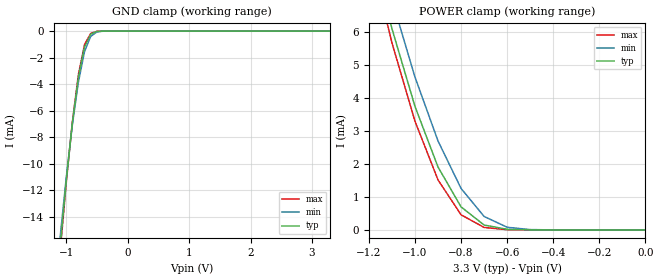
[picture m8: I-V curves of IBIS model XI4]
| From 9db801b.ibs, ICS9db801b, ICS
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|   Model XI4
[Model]   XI4
Model_type   Input
Polarity   Non-Inverting
Vinl =   0.175V
Vinh =   0.525V
C_comp   3.40pF   2.85pF   3.95pF
[Temperature Range]   25.00   71.00   1.00
[Voltage Range]   3.30V   3.00V   3.70V
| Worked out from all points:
|   GND clamp passes 1 mA (typ) near -0.68 V on its own axis
|   POWER clamp passes 1 mA (typ) near -0.82 V on its own axis
[GND_clamp]
| voltage   I(typ)   I(min)   I(max)
-3.3V     -160mA     -150mA     -160mA
-1.1V     -16.38mA   -15.67mA   -16.85mA
-1V       -11.38mA   -11.14mA   -11.54mA
-900mV    -6.99mA    -7.13mA    -6.92mA
-800mV    -3.48mA    -3.84mA    -3.27mA
-700mV    -1.2mA     -1.54mA    -1.01mA
-600mV    -240uA     -400uA     -170uA
-500mV    -29.28uA   -66.42uA   -17.31uA
-400mV    -2.53uA    -8.31uA    -1.16uA
3.3V      160pA      130nA      110pA
[POWER_clamp]
| voltage   I(typ)   I(min)   I(max)
-3.3V     130mA      120mA      140mA
-1.2V     8.92mA     9.69mA     8.55mA
-1.1V     6.11mA     6.99mA     5.68mA
-1V       3.75mA     4.64mA     3.3mA
-900mV    1.91mA     2.7mA      1.52mA
-800mV    700uA      1.26mA     460uA
-700mV    150uA      410uA      77.11uA
-600mV    19.94uA    82.32uA    8.03uA
-500mV    1.95uA     11.93uA    590nA
0V        160pA      550pA      150pA
